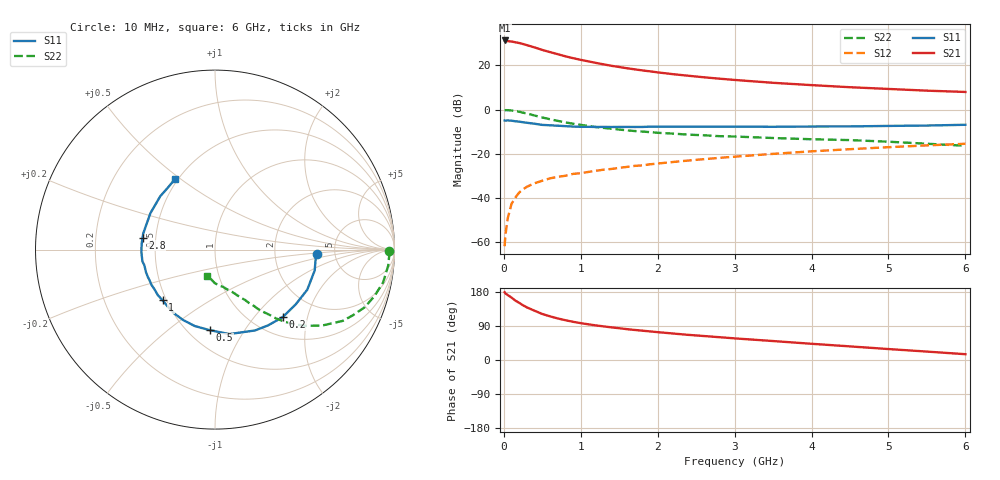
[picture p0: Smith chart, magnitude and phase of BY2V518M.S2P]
! SIEMENS Small Signal Semiconductors
! BFY420
! Si NPN RF SIEGET Grounded Emitter Transistor in MICRO-X
! VCE = 2.5 V  IC = 18 mA
! Common Emitter S-Parameters:  October  1996
# GHz  S  MA  R  50
!  f  S11  S21  S12  S22
! GHz  MAG  ANG  MAG  ANG  MAG  ANG  MAG  ANG
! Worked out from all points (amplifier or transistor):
!   36 points, 10 MHz to 6 GHz, reference 50 ohm
!   highest |S21| = 31.3 dB at 10 MHz (marker M1)
!   |S21| within 3 dB of that: start of sweep to 383.9 MHz
!   unconditionally stable (mu >= 1): 2.039 GHz to end of sweep
!   at 250 MHz: K = 0.28, MSG = 33.0 dB, |S12| = -36.2 dB
!   at 1.4 GHz: K = 0.89, MSG = 23.4 dB, |S12| = -26.9 dB
!   at 6 GHz: K = 1.07, MAG = 10.1 dB, |S12| = -15.5 dB
!   S11 on the Smith chart (normalised r, x): 10 MHz: 3.60, -0.26; 200 MHz: 1.35, -1.42; 500 MHz: 0.63, -0.71; 1 GHz: 0.48, -0.32; 2.8 GHz: 0.42, +0.07; 6 GHz: 0.48, +0.48
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0.01  0.5672 -2.5  36.94 178.7  0.0008 101.2  0.9667 -0.6
0.02  0.5632 -5.1  36.6 175.8  0.0014 89.4  0.9714 -1.8
0.1  0.5606 -23.5  34.96 164.7  0.0073 80.8  0.9542 -11.1
0.15  0.5435 -34.1  33.56 156.7  0.0101 75.7  0.925 -16.3
0.2  0.5328 -44.9  32.31 150.8  0.0132 72.7  0.8943 -21.0
0.25  0.5157 -54.9  30.64 144.3  0.0155 68.7  0.8517 -25.4
0.3  0.5026 -63.7  28.92 138.8  0.0178 66.8  0.8143 -29.2
0.4  0.4774 -80.3  25.65 129.9  0.0214 62.9  0.7332 -35.2
0.5  0.4499 -93.7  22.51 121.4  0.0244 59.5  0.6627 -39.9
0.6  0.4405 -104.9  20.13 115.2  0.0276 58.3  0.6037 -43.5
0.7  0.4305 -114.4  18.05 109.7  0.0298 57.3  0.5552 -46.2
0.8  0.4218 -123.0  16.15 105.0  0.0316 55.4  0.5129 -48.4
1  0.4063 -136.0  13.42 97.3  0.0362 56.8  0.45 -51.5
1.1  0.4071 -141.6  12.38 94.1  0.0386 56.9  0.4249 -53.2
1.4  0.4027 -155.0  9.82 86.1  0.0451 56.8  0.3685 -56.3
1.6  0.4045 -162.0  8.65 81.4  0.0501 56.3  0.3383 -58.4
2.2  0.4101 -177.6  6.348 69.9  0.0649 54.8  0.2851 -63.9
2.8  0.4089 170.6  5.027 60.2  0.0803 52.6  0.2497 -68.6
3.5  0.4072 158.4  4.047 50.0  0.0991 48.2  0.2267 -74.2
4.5  0.4159 143.1  3.215 35.9  0.1265 40.7  0.2033 -82.7
5.5  0.4347 126.6  2.686 22.2  0.1542 31.8  0.1681 -96.8
6  0.4525 119.4  2.511 15.3  0.1678 27.0  0.1514 -106.7
